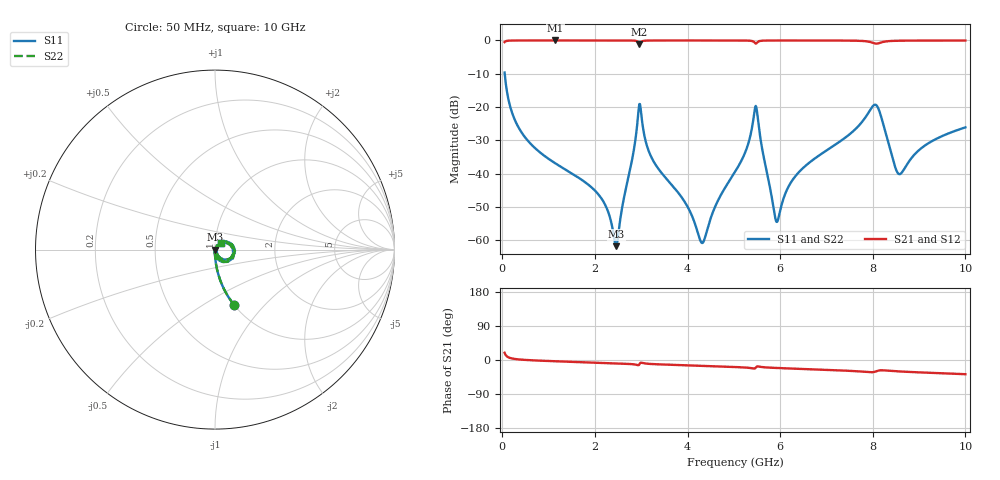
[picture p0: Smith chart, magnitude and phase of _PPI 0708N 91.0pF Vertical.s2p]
! S-Parameter data specifications (vertical orientation):
! Substrate: 40-mil Rogers 3003C, Substrate thickness, H=1.016mm, Dielectric constant, Er=3, Conductor thickness, T_mtl=0.043mm, Loss Tangent, Tand=0.003
! PCB Mounting Pad Footprint: Pad width, PadW=2.54mm , Pad length, PadL=0.51mm , Pad gap, PadG (edge-to-edge)=0.71mm , Reference planes=1.73mm apart
! Created Tue Jan 16 08:54:33 2018
# GHz S MA R 50
! 2 Port Network Data from SP1.SP block
! freq  magS11  angS11  magS21  angS21  magS12  angS12  magS22  angS22
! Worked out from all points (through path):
!   801 points, 50 MHz to 10 GHz, reference 50 ohm
!   highest |S21| = 0.00 dB at 1.145 GHz (marker M1); lowest = -1.0 dB at 2.96 GHz (marker M2)
!   group delay of S21, straight-line fit = 10.8 ps
!   lowest |S11| = -61.8 dB at 2.463 GHz (marker M3), VSWR 1.00, Z = 50.1 - j0.0091 ohm
!   |S11| at or under -10 dB: 52.51 MHz to end of sweep
!   |S22| runs from -61.8 to -9.6 dB; largest |S21 - S12| = 0
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0.05  0.3294 -70.9  0.944 19.1  0.944 19.1  0.3294 -70.9
0.373375  0.04646 -88.4  0.9987 1.3  0.9987 1.3  0.04646 -88.4
1.1445  0.01432 -91.8  0.9995 -3.3  0.9995 -3.3  0.01432 -91.8
1.716625  0.008081 -92.4  0.9994 -5.7  0.9994 -5.7  0.008081 -92.4
2.18925  0.003754 -88.5  0.9993 -7.7  0.9993 -7.7  0.003754 -88.5
2.462875  0.0008172 -6.4  0.9991 -8.9  0.9991 -8.9  0.0008172 -6.4
2.960375  0.1114 -3.8  0.8894 -11.5  0.8894 -11.5  0.1114 -3.8
3.146937  0.02336 -90.4  0.9957 -10.0  0.9957 -10.0  0.02336 -90.4
3.370812  0.01185 -94.6  0.9984 -11.4  0.9984 -11.4  0.01185 -94.6
3.955375  0.003623 -89.6  0.9989 -14.0  0.9989 -14.0  0.003623 -89.6
4.316063  0.0009101 -16.3  0.9989 -15.4  0.9989 -15.4  0.0009101 -16.3
5.025  0.01064 63.3  0.9982 -18.5  0.9982 -18.5  0.01064 63.3
5.27375  0.02355 59.5  0.9953 -20.1  0.9953 -20.1  0.02355 59.5
5.47275  0.1041 -13.2  0.8964 -20.2  0.8964 -20.2  0.1041 -13.2
5.9205  0.001895 -21.7  0.9979 -21.0  0.9979 -21.0  0.001895 -21.7
6.231438  0.007375 55.9  0.9982 -22.5  0.9982 -22.5  0.007375 55.9
6.691625  0.01582 59.5  0.998 -24.6  0.998 -24.6  0.01582 59.5
8.034875  0.1081 -0.2  0.9056 -31.4  0.9056 -31.4  0.1081 -0.2
8.345812  0.02754 -62.5  0.9767 -28.3  0.9767 -28.3  0.02754 -62.5
8.594563  0.009912 -0.4  0.991 -30.3  0.991 -30.3  0.009912 -0.4
9.116938  0.02621 49.0  0.9957 -33.2  0.9957 -33.2  0.02621 49.0
10  0.04958 49.9  0.9961 -37.5  0.9961 -37.5  0.04958 49.9
